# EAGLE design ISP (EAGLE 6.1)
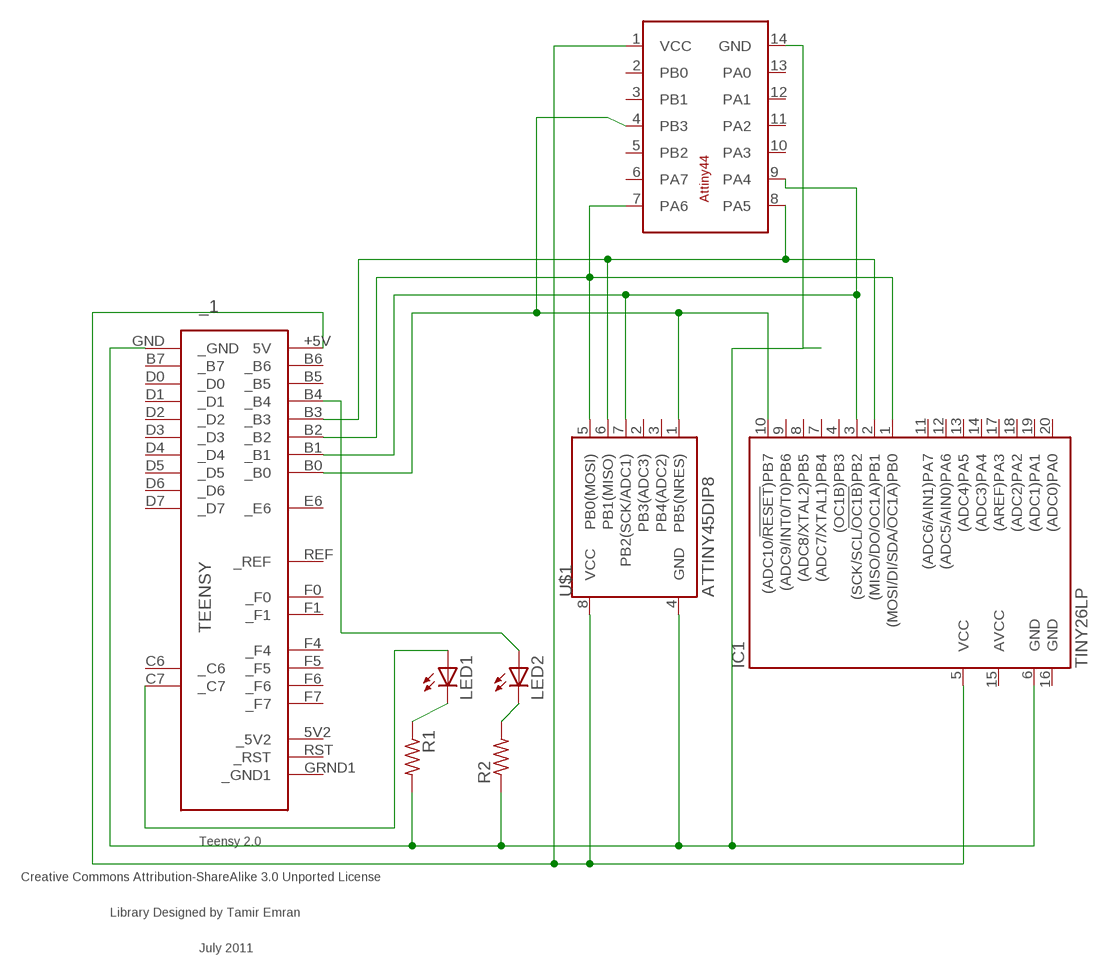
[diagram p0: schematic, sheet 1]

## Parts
_1  TEENSY  [TEENSY]
IC1  TINY26LP  [DIL20]
LED1  LED3MM  [LED3MM]
LED2  LED3MM  [LED3MM]
R1  R-US_0204/5  [0204/5]
R2  R-US_0204/5  [0204/5]
U$1  ATTINY45DIP8  [DIP08]
U$2  ATTINY44-DIL14  [DIL14]

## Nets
5V: _1.+5V(5V) IC1.5(VCC) U$1.8(VCC) U$2.1(VCC)
GROUND: _1.GND(_GND) IC1.6(GND) R1.2 R2.1 U$1.4(GND) U$2.14(GND)
MISO: _1.B3(_B3) IC1.2((MISO/DO/OC1A)PB1) U$1.6(PB1(MISO)) U$2.8(PA5)
MOSI: _1.B2(_B2) IC1.1((MOSI/DI/SDA/!OC1A!)PB0) U$1.5(PB0(MOSI)) U$2.7(PA6)
N$3: LED1.K(C) R1.1
N$4: LED2.K(C) R2.2
N$5: _1.C7(_C7) LED1.A
N$6: _1.B4(_B4) LED2.A
RESET: _1.B0(_B0) IC1.10((ADC10/!RESET!)PB7) U$1.1(PB5(NRES)) U$2.4(PB3)
SCK: _1.B1(_B1) IC1.3((SCK/SCL/!OC1B!)PB2) U$1.7(PB2(SCK/ADC1)) U$2.9(PA4)
Unconnected: _1.5V2(_5V2) _1.B5(_B5) _1.B6(_B6) _1.B7(_B7) _1.C6(_C6) _1.D0(_D0) _1.D1(_D1) _1.D2(_D2) _1.D3(_D3) _1.D4(_D4) _1.D5(_D5) _1.D6(_D6) _1.D7(_D7) _1.E6(_E6) _1.F0(_F0) _1.F1(_F1) _1.F4(_F4) _1.F5(_F5) _1.F6(_F6) _1.F7(_F7) _1.GRND1(_GND1) _1.REF(_REF) _1.RST(_RST) IC1.4((OC1B)PB3) IC1.7((ADC7/XTAL1)PB4) IC1.8((ADC8/XTAL2)PB5) IC1.9((ADC9/INT0/T0)PB6) IC1.11((ADC6/AIN1)PA7) IC1.12((ADC5/AIN0)PA6) IC1.13((ADC4)PA5) IC1.14((ADC3)PA4) IC1.17((AREF)PA3) IC1.18((ADC2)PA2) IC1.19((ADC1)PA1) IC1.20((ADC0)PA0) U$1.2(PB3(ADC3)) U$1.3(PB4(ADC2)) U$2.2(PB0) U$2.3(PB1) U$2.5(PB2) U$2.6(PA7) U$2.10(PA3) U$2.11(PA2) U$2.12(PA1) U$2.13(PA0)

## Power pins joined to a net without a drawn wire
AVCC: IC1.15(AVCC)
GND: IC1.16(GND)

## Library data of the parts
_1 = teensy:TEENSY: Teensy 2.0 Original Design by Clint Fisher Modified Design by Tamir Emran Licensed Under Creative Commons Attribution-ShareAlike 3.0 Unported (CC BY-SA 3.0)
IC1 = atmel:TINY26*: 8-bit AVR Microcontroller with 2K Bytes Flash Source: http://www.atmel.com .. doc1477.pdf; MPN: ATTINY26L-8PU; OC_FARNELL: 9171657; OC_NEWARK: 01M6920
LED1 LED2 = adafruit:LED: LED
R1 R2 = adafruit:R-US_: RESISTOR, American symbol
U$1 = SparkFun:ATTINY45: Atmel ATTiny45
U$2 = atmel-new:ATTINY44-DIL14

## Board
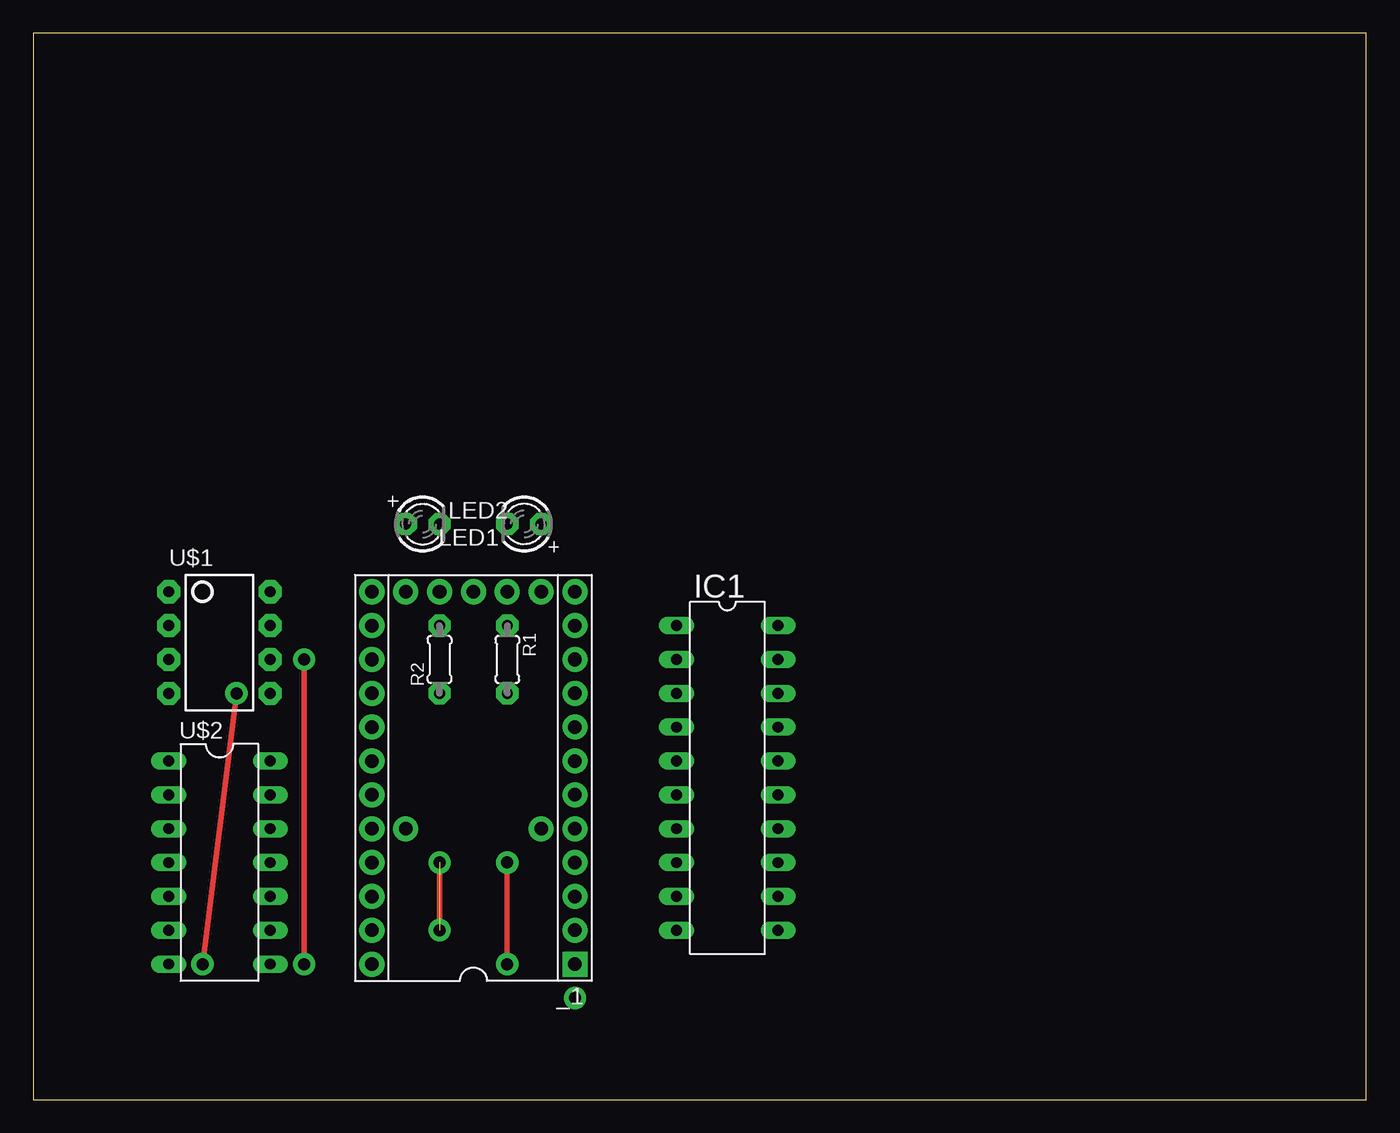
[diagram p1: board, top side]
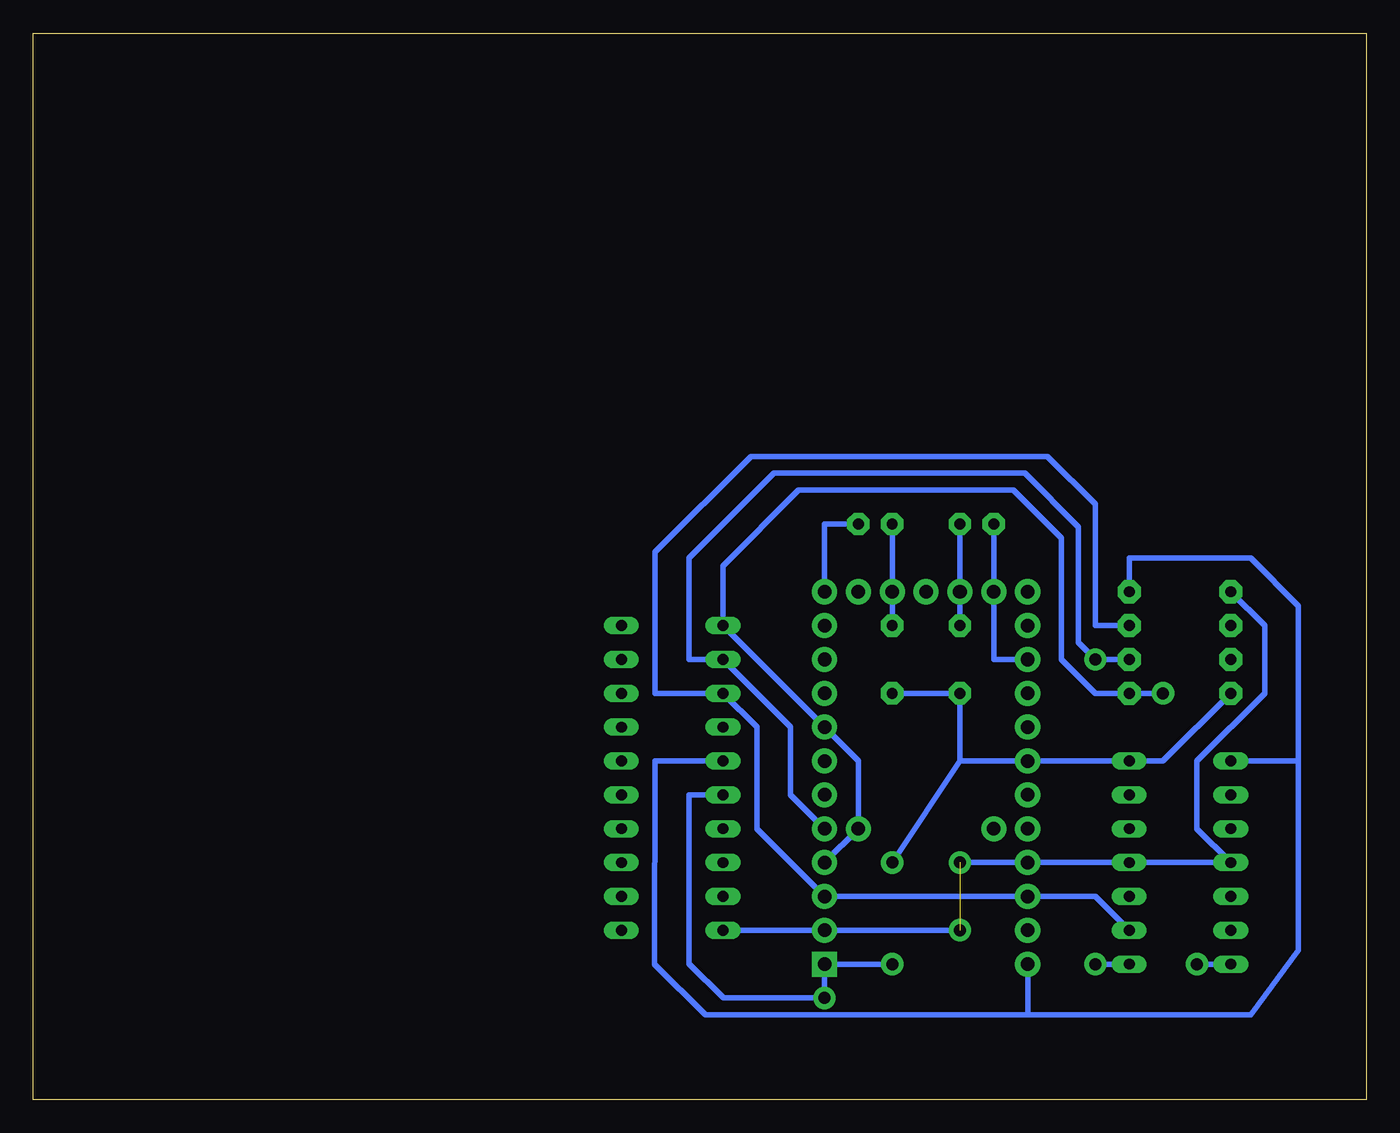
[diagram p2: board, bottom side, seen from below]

Size 100 x 80 mm. Coordinates in mm from the lower left corner, seen from the top.
Outline: 0,0 100,0 100,80 0,80 0,0
Copper layers (1*16): Top 0.035mm / dielectric 1.5mm / Bottom 0.035mm
Design rules: minimum track width 10mil, minimum drill 24mil, track to track 8mil, track to pad 8mil, pad to pad 8mil, via to via 8mil, smd to smd 8mil, copper to edge 40mil, drill to drill 8mil, minimum pad ring 10mil, minimum via ring 8mil, stop-mask expansion 4mil, vias tented up to drill 0mil, thermal gap 10mil

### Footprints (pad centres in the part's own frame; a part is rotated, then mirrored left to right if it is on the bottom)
TEENSY = drill 1.016 pad 1.88: 5V2 13.97,-2.54; +5V -13.97,7.62; B0 -11.43,-7.62; B1 -8.89,-7.62; B2 -6.35,-7.62; B3 -3.81,-7.62; B4 8.89,7.62; B5 6.35,7.62; B6 3.81,7.62; B7 -1.27,-7.62; C6 11.43,-7.62; C7 13.97,-7.62; D0 1.27,-7.62; D1 3.81,-7.62; D2 6.35,-7.62; D3 8.89,-7.62; D4 13.97,5.08; D5 13.97,-5.08; D6 13.97,7.62; D7 11.43,7.62; E6 -3.81,-5.08; F0 -11.43,7.62; F1 -8.89,7.62; F4 -6.35,7.62; F5 -3.81,7.62; F6 -1.27,7.62; F7 1.27,7.62; GRND1 13.97,0; REF -3.81,5.08; RST 13.97,2.54 | drill 1.016 pad 1.88 square: GND -13.97,-7.62
DIL20 = drill 0.813 long: 1 -11.43,-3.81; 2 -8.89,-3.81; 3 -6.35,-3.81; 4 -3.81,-3.81; 5 -1.27,-3.81; 6 1.27,-3.81; 7 3.81,-3.81; 8 6.35,-3.81; 9 8.89,-3.81; 10 11.43,-3.81; 11 11.43,3.81; 12 8.89,3.81; 13 6.35,3.81; 14 3.81,3.81; 15 1.27,3.81; 16 -1.27,3.81; 17 -3.81,3.81; 18 -6.35,3.81; 19 -8.89,3.81; 20 -11.43,3.81
LED3MM = drill 0.813 pad 1.676 octagon: A -1.27,0; K 1.27,0
0204/5 = drill 0.813 pad 1.676 octagon: 1 -2.54,0; 2 2.54,0
DIP08 = drill 0.813 pad 1.727 octagon: 1 -3.81,-3.81; 2 -1.27,-3.81; 3 1.27,-3.81; 4 3.81,-3.81; 5 3.81,3.81; 6 1.27,3.81; 7 -1.27,3.81; 8 -3.81,3.81
DIL14 = drill 0.813 long: 1 -7.62,-3.81; 2 -5.08,-3.81; 3 -2.54,-3.81; 4 0,-3.81; 5 2.54,-3.81; 6 5.08,-3.81; 7 7.62,-3.81; 8 7.62,3.81; 9 5.08,3.81; 10 2.54,3.81; 11 0,3.81; 12 -2.54,3.81; 13 -5.08,3.81; 14 -7.62,3.81

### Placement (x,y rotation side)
_1  33.02,24.13 90 top
IC1  52.07,24.13 270 top
LED1  36.83,43.18 180 top
LED2  29.21,43.18 0 top
R1  35.56,33.02 270 top
R2  30.48,33.02 90 top
U$1  13.97,34.29 270 top
U$2  13.97,17.78 270 top

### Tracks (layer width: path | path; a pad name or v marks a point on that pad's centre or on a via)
5V
  Bottom 0.406: 25.4,6.35 8.67,6.35 5.08,11.21 5.08,25.4 | 5.08,25.4 5.08,37.05 8.67,40.64 17.78,40.64 U$1.8 | _1.+5V 25.4,6.35 | 25.4,6.35 49.56,6.35 53.38,10.16 53.34,25.4 IC1.5 | U$2.1 5.08,25.4
GROUND  (via drill 0.9 pad 1.68)
  Top 0.406: v35.56,10.16 v35.56,17.78
  Bottom 0.406: IC1.6 50.8,22.86 50.8,10.2 48.22,7.62 v40.64,7.62 _1.GND v35.56,10.16 | R1.2 R2.1 30.48,25.4 | 30.48,25.4 U$2.14 15.24,25.4 U$1.4 | v35.56,17.78 30.48,25.4
MISO  (via drill 0.9 pad 1.68)
  Top 0.406: v20.32,33.02 v20.32,10.16
  Bottom 0.406: _1.B3 43.18,22.86 43.18,27.94 IC1.2 50.8,33.02 50.8,40.64 44.45,46.99 25.61,46.99 21.59,42.97 21.59,34.29 v20.32,33.02 U$1.6 | U$2.8 v20.32,10.16
MOSI  (via drill 0.9 pad 1.68)
  Top 0.406: v15.24,30.48 v12.7,10.16
  Bottom 0.406: _1.B2 38.1,20.32 38.1,25.4 IC1.1 48.26,40.04 42.58,45.72 26.45,45.72 22.86,42.13 22.86,33.02 20.32,30.48 U$1.5 v15.24,30.48 | U$2.7 v12.7,10.16
N$3
  Bottom 0.406: LED1.K R1.1
N$4
  Bottom 0.406: LED2.K R2.2
N$5
  Bottom 0.406: LED1.A 40.64,43.18 _1.C7
N$6
  Bottom 0.406: _1.B4 27.94,33.02 LED2.A
N$8  (via drill 0.9 pad 1.68)
  Top 0.406: v30.48,12.7 v30.48,17.78
RESET  (1 unrouted)
  Bottom 0.406: IC1.10 _1.B0 30.48,12.7 | 30.48,17.78 U$2.4 12.7,20.32 12.7,25.4 7.62,30.48 7.62,35.56 U$1.1
SCK
  Bottom 0.406: U$2.9 20.32,15.24 _1.B1 45.72,20.32 45.72,27.94 IC1.3 53.34,30.48 53.34,41.08 46.16,48.26 23.91,48.26 20.32,44.67 20.32,35.56 U$1.7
